| TEXAS INSTRUMENTS INCORPORATED
| Standard Linear and Logic Group
| IBIS Model of SN74ALVCH16646
| 16 BIT BUS TRANSCEIVER AND REGISTER WITH 3-STATE OUTPUTS
| This file contains package information for the following:
|  SSOP 56-pin (DL) package as [Component] ALVCH16646_DL
|  TSSOP 56-pin (DGG) package as [Component] ALVCH16646_DGG
|  TVSOP 56-pin (DGV) package as [Component] ALVCH16646_DGV
| This device can be powered at the following Vccs:
|  2.5 volt Vcc
|  3.3 volt Vcc
|  1.8 volt Vcc
| This file provides unique models under the [Model Selector] for each Vcc.
| For operation at a specific Vcc, select the appropriate model after each
| [Model Selector] keyword.
[IBIS Ver]   3.2
[Comment char]  |_char
[File Name]   sn74alvch16646.ibs
[File Rev]   1.1 | a_die
[Date]   October 1, 2001
[Source]   Data created from TI-SPICE simulations at TI-SLL.
[Notes]   The following is an IBIS list for the ALVCH16646.
   Please contact sllibis@ti.com with questions and
   comments concerning SLL IBIS models.
   This IBIS model is created from a BA (back annotated netlist
   Non-Convergence in the following files:
   gc_alvch16646_noe_33, extrapolated from 0.5 V plus
   gc_alvch16646_dir_25, extrapolated from 0.525 V plus
   Non-Convergence in the following files:
[Disclaimer] Property of Texas Instruments Incorporated.  Unauthorized
   reproduction and/or distribution is strictly prohibited.
   This product is protected under copyright law.
   Created  2001, (C) Copyright  2001, Texas Instruments
   Incorporated, All Rights Reserved
   UNLESS THERE IS A SIGNED, WRITTEN AGREEMENT TO THE
   CONTRARY, TEXAS INSTRUMENTS (TI) IS PROVIDING THE IBIS
   MODELS  AND WITHOUT ANY WARRANTY, EXPRESSED OR
   IMPLIED.  TI assumes no liability for:
   1) the accuracy of the IBIS models provided to your
   company;
   2) the proper functioning of these IBIS Models in your
   design or for any resulting applications; or
   3) infringement of patents, copyrights or intellectual
   property rights resulting from your use of these IBIS
   models.
   TI provides IBIS Models as a service to our customers.
   You and your company shall not distribute, sell or give
   these models to anyone else without prior written
   permission from TI.
   TI reserves the right to make changes to our products or
   to discontinue any semiconductor product or service
   without notice, and advises our customers to obtain the
   latest version of relevant information to verify, before
   placing orders, that the information being relied on is
   current.
   Please be aware that your receipt and use of the IBIS
   information provided shall serve as acceptance of these
   terms and conditions.  If you do not accept these terms,
   you should return or destroy the IBIS models and any
   other accompanying information immediately.
| Component ALVCH16646_DL 56-pin SSOP
[Component]   ALVCH16646_DL
[Manufacturer]   Texas Instruments, Inc.
[Package]
|   typ   min   max
R_pkg   5.500e-02   4.800e-02   6.700e-02
L_pkg   6.539e-09   4.802e-09   9.746e-09
C_pkg   1.880e-13   7.600e-14   5.170e-13
[Pin]   signal_name   model_name   R_pin   L_pin   C_pin
1   1DIR   ALVCH16646_DIR   6.400e-02   9.646e-09   5.130e-13
2   1CLKAB   ALVCH16646_CLK   5.900e-02   8.723e-09   2.700e-13
3   1SAB   ALVCH16646_STORE   5.900e-02   8.139e-09   2.230e-13
4   GND   GND   5.600e-02   7.554e-09   2.010e-13
5   1A1   ALVCH16646_IO   5.400e-02   6.991e-09   1.950e-13
6   1A2   ALVCH16646_IO   5.300e-02   6.659e-09   2.020e-13
7   VCC   POWER   5.500e-02   6.321e-09   2.070e-13
8   1A3   ALVCH16646_IO   5.500e-02   5.942e-09   1.330e-13
9   1A4   ALVCH16646_IO   5.700e-02   5.767e-09   1.320e-13
10   1A5   ALVCH16646_IO   5.400e-02   5.459e-09   1.210e-13
11   GND   GND   5.100e-02   5.224e-09   1.400e-13
12   1A6   ALVCH16646_IO   4.800e-02   5.088e-09   1.260e-13
13   1A7   ALVCH16646_IO   5.000e-02   5.021e-09   9.600e-14
14   1A8   ALVCH16646_IO   5.100e-02   4.802e-09   7.600e-14
15   2A1   ALVCH16646_IO   5.100e-02   4.803e-09   7.600e-14
16   2A2   ALVCH16646_IO   5.000e-02   5.021e-09   9.600e-14
17   2A3   ALVCH16646_IO   4.800e-02   5.088e-09   1.260e-13
18   GND   GND   5.100e-02   5.224e-09   1.400e-13
19   2A4   ALVCH16646_IO   5.400e-02   5.459e-09   1.210e-13
20   2A5   ALVCH16646_IO   5.700e-02   5.768e-09   1.330e-13
21   2A6   ALVCH16646_IO   5.500e-02   5.942e-09   1.330e-13
22   VCC   POWER   5.500e-02   6.320e-09   2.060e-13
23   2A7   ALVCH16646_IO   5.300e-02   6.659e-09   2.030e-13
24   2A8   ALVCH16646_IO   5.400e-02   6.991e-09   1.960e-13
25   GND   GND   5.600e-02   7.554e-09   2.010e-13
26   2SAB   ALVCH16646_STORE   5.900e-02   8.139e-09   2.230e-13
27   2CLKAB   ALVCH16646_CLK   5.900e-02   8.727e-09   2.700e-13
28   2DIR   ALVCH16646_DIR   6.700e-02   9.746e-09   5.170e-13
29   2NOE   ALVCH16646_NOE   6.300e-02   9.630e-09   5.110e-13
30   2CLKBA   ALVCH16646_CLK   6.000e-02   8.751e-09   2.710e-13
31   2SBA   ALVCH16646_STORE   6.000e-02   8.184e-09   2.250e-13
32   GND   GND   5.600e-02   7.543e-09   2.000e-13
33   2B8   ALVCH16646_IO   5.400e-02   7.005e-09   1.960e-13
34   2B7   ALVCH16646_IO   5.600e-02   6.714e-09   2.040e-13
35   VCC   POWER   5.800e-02   6.384e-09   2.080e-13
36   2B6   ALVCH16646_IO   5.700e-02   5.976e-09   1.340e-13
37   2B5   ALVCH16646_IO   5.700e-02   5.743e-09   1.300e-13
38   2B4   ALVCH16646_IO   5.400e-02   5.468e-09   1.190e-13
39   GND   GND   5.500e-02   5.328e-09   1.420e-13
40   2B3   ALVCH16646_IO   5.200e-02   5.189e-09   1.290e-13
41   2B2   ALVCH16646_IO   5.200e-02   5.053e-09   9.600e-14
42   2B1   ALVCH16646_IO   5.100e-02   4.825e-09   7.600e-14
43   1B8   ALVCH16646_IO   5.400e-02   4.896e-09   7.800e-14
44   1B7   ALVCH16646_IO   5.200e-02   5.093e-09   9.700e-14
45   1B6   ALVCH16646_IO   5.100e-02   5.179e-09   1.280e-13
46   GND   GND   5.400e-02   5.314e-09   1.420e-13
47   1B5   ALVCH16646_IO   5.500e-02   5.511e-09   1.210e-13
48   1B4   ALVCH16646_IO   5.700e-02   5.771e-09   1.310e-13
49   1B3   ALVCH16646_IO   5.600e-02   5.957e-09   1.330e-13
50   VCC   POWER   5.500e-02   6.320e-09   2.060e-13
51   1B2   ALVCH16646_IO   5.200e-02   6.621e-09   2.000e-13
52   1B1   ALVCH16646_IO   5.300e-02   6.973e-09   1.950e-13
53   GND   GND   5.700e-02   7.571e-09   2.020e-13
54   1SBA   ALVCH16646_STORE   5.700e-02   8.097e-09   2.220e-13
55   1CLKBA   ALVCH16646_CLK   5.900e-02   8.723e-09   2.710e-13
56   1NOE   ALVCH16646_NOE   6.100e-02   9.560e-09   5.090e-13
| Component ALVCH16646_DGG 56-pin TSSOP
[Component]   ALVCH16646_DGG
[Manufacturer]   Texas Instruments, Inc.
[Package]
|   typ   min   max
R_pkg   4.500e-02   3.500e-02   6.200e-02
L_pkg   3.324e-09   2.403e-09   5.094e-09
C_pkg   5.640e-13   3.410e-13   9.140e-13
[Pin]   signal_name   model_name   R_pin   L_pin   C_pin
1   1DIR   ALVCH16646_DIR   6.200e-02   5.094e-09   8.560e-13
2   1CLKAB   ALVCH16646_CLK   6.100e-02   4.621e-09   9.020e-13
3   1SAB   ALVCH16646_STORE   6.000e-02   4.316e-09   8.020e-13
4   GND   GND   5.900e-02   3.968e-09   6.980e-13
5   1A1   ALVCH16646_IO   5.700e-02   3.716e-09   6.490e-13
6   1A2   ALVCH16646_IO   4.200e-02   3.517e-09   6.520e-13
7   VCC   POWER   4.100e-02   3.160e-09   5.700e-13
8   1A3   ALVCH16646_IO   3.900e-02   2.981e-09   4.820e-13
9   1A4   ALVCH16646_IO   3.900e-02   2.809e-09   4.470e-13
10   1A5   ALVCH16646_IO   3.800e-02   2.715e-09   4.090e-13
11   GND   GND   4.100e-02   2.675e-09   3.910e-13
12   1A6   ALVCH16646_IO   3.900e-02   2.536e-09   3.660e-13
13   1A7   ALVCH16646_IO   3.900e-02   2.457e-09   3.480e-13
14   1A8   ALVCH16646_IO   3.800e-02   2.411e-09   3.530e-13
15   2A1   ALVCH16646_IO   3.900e-02   2.456e-09   3.550e-13
16   2A2   ALVCH16646_IO   3.900e-02   2.471e-09   3.490e-13
17   2A3   ALVCH16646_IO   4.000e-02   2.580e-09   3.700e-13
18   GND   GND   3.800e-02   2.651e-09   3.890e-13
19   2A4   ALVCH16646_IO   3.800e-02   2.739e-09   4.110e-13
20   2A5   ALVCH16646_IO   3.900e-02   2.838e-09   4.490e-13
21   2A6   ALVCH16646_IO   3.800e-02   2.988e-09   4.840e-13
22   VCC   POWER   3.800e-02   3.105e-09   5.640e-13
23   2A7   ALVCH16646_IO   4.000e-02   3.427e-09   6.380e-13
24   2A8   ALVCH16646_IO   5.600e-02   3.654e-09   6.410e-13
25   GND   GND   5.700e-02   3.932e-09   7.000e-13
26   2SAB   ALVCH16646_STORE   5.800e-02   4.257e-09   8.060e-13
27   2CLKAB   ALVCH16646_CLK   5.700e-02   4.580e-09   9.140e-13
28   2DIR   ALVCH16646_DIR   5.900e-02   5.038e-09   8.610e-13
29   2NOE   ALVCH16646_NOE   6.000e-02   5.058e-09   8.580e-13
30   2CLKBA   ALVCH16646_CLK   5.600e-02   4.543e-09   9.040e-13
31   2SBA   ALVCH16646_STORE   5.700e-02   4.240e-09   8.030e-13
32   GND   GND   5.700e-02   3.929e-09   7.000e-13
33   2B8   ALVCH16646_IO   5.600e-02   3.616e-09   6.370e-13
34   2B7   ALVCH16646_IO   3.700e-02   3.368e-09   6.400e-13
35   VCC   POWER   3.600e-02   3.024e-09   5.630e-13
36   2B6   ALVCH16646_IO   3.500e-02   2.876e-09   4.740e-13
37   2B5   ALVCH16646_IO   3.500e-02   2.745e-09   4.440e-13
38   2B4   ALVCH16646_IO   3.700e-02   2.683e-09   4.050e-13
39   GND   GND   3.800e-02   2.603e-09   3.820e-13
40   2B3   ALVCH16646_IO   3.800e-02   2.510e-09   3.620e-13
41   2B2   ALVCH16646_IO   3.600e-02   2.412e-09   3.410e-13
42   2B1   ALVCH16646_IO   3.800e-02   2.416e-09   3.490e-13
43   1B8   ALVCH16646_IO   3.700e-02   2.403e-09   3.490e-13
44   1B7   ALVCH16646_IO   3.700e-02   2.429e-09   3.410e-13
45   1B6   ALVCH16646_IO   3.600e-02   2.482e-09   3.580e-13
46   GND   GND   3.700e-02   2.615e-09   3.810e-13
47   1B5   ALVCH16646_IO   3.500e-02   2.669e-09   4.020e-13
48   1B4   ALVCH16646_IO   3.600e-02   2.763e-09   4.420e-13
49   1B3   ALVCH16646_IO   3.600e-02   2.942e-09   4.780e-13
50   VCC   POWER   3.500e-02   3.053e-09   5.640e-13
51   1B2   ALVCH16646_IO   3.600e-02   3.409e-09   6.410e-13
52   1B1   ALVCH16646_IO   5.800e-02   3.698e-09   6.410e-13
53   GND   GND   5.900e-02   3.975e-09   6.970e-13
54   1SBA   ALVCH16646_STORE   6.100e-02   4.327e-09   8.020e-13
55   1CLKBA   ALVCH16646_CLK   6.100e-02   4.624e-09   9.050e-13
56   1NOE   ALVCH16646_NOE   6.000e-02   5.063e-09   8.580e-13
| Component ALVCH16646_DGV 56-pin TVSOP
[Component]   ALVCH16646_DGV
[Manufacturer]   Texas Instruments, Inc.
[Package]
|   typ   min   max
R_pkg   6.300e-02   5.000e-02   8.600e-02
L_pkg   2.945e-09   2.392e-09   3.938e-09
C_pkg   3.910e-13   2.710e-13   5.880e-13
[Pin]   signal_name   model_name   R_pin   L_pin   C_pin
1   1DIR   ALVCH16646_DIR   6.800e-02   3.933e-09   5.880e-13
2   1CLKAB   ALVCH16646_CLK   6.800e-02   3.569e-09   5.860e-13
3   1SAB   ALVCH16646_STORE   7.600e-02   3.464e-09   5.150e-13
4   GND   GND   8.600e-02   3.451e-09   4.580e-13
5   1A1   ALVCH16646_IO   8.200e-02   3.278e-09   4.260e-13
6   1A2   ALVCH16646_IO   7.700e-02   3.143e-09   3.870e-13
7   VCC   POWER   6.900e-02   2.971e-09   4.010e-13
8   1A3   ALVCH16646_IO   5.000e-02   2.787e-09   3.790e-13
9   1A4   ALVCH16646_IO   5.100e-02   2.686e-09   3.200e-13
10   1A5   ALVCH16646_IO   5.200e-02   2.607e-09   3.160e-13
11   GND   GND   5.300e-02   2.497e-09   2.970e-13
12   1A6   ALVCH16646_IO   5.400e-02   2.438e-09   2.920e-13
13   1A7   ALVCH16646_IO   5.500e-02   2.412e-09   2.860e-13
14   1A8   ALVCH16646_IO   5.500e-02   2.400e-09   2.730e-13
15   2A1   ALVCH16646_IO   5.500e-02   2.402e-09   2.730e-13
16   2A2   ALVCH16646_IO   5.400e-02   2.398e-09   2.840e-13
17   2A3   ALVCH16646_IO   5.400e-02   2.407e-09   2.890e-13
18   GND   GND   5.300e-02   2.448e-09   2.930e-13
19   2A4   ALVCH16646_IO   5.200e-02   2.548e-09   3.110e-13
20   2A5   ALVCH16646_IO   5.100e-02   2.623e-09   3.160e-13
21   2A6   ALVCH16646_IO   5.000e-02   2.725e-09   3.700e-13
22   VCC   POWER   6.500e-02   2.903e-09   3.940e-13
23   2A7   ALVCH16646_IO   7.300e-02   3.086e-09   3.870e-13
24   2A8   ALVCH16646_IO   8.200e-02   3.272e-09   4.280e-13
25   GND   GND   8.200e-02   3.394e-09   4.570e-13
26   2SAB   ALVCH16646_STORE   7.100e-02   3.374e-09   5.080e-13
27   2CLKAB   ALVCH16646_CLK   6.900e-02   3.572e-09   5.810e-13
28   2DIR   ALVCH16646_DIR   6.900e-02   3.937e-09   5.740e-13
29   2NOE   ALVCH16646_NOE   6.900e-02   3.923e-09   5.690e-13
30   2CLKBA   ALVCH16646_CLK   6.800e-02   3.546e-09   5.740e-13
31   2SBA   ALVCH16646_STORE   7.400e-02   3.422e-09   5.180e-13
32   GND   GND   8.100e-02   3.395e-09   4.680e-13
33   2B8   ALVCH16646_IO   8.000e-02   3.255e-09   4.310e-13
34   2B7   ALVCH16646_IO   7.100e-02   3.063e-09   3.860e-13
35   VCC   POWER   6.100e-02   2.878e-09   3.900e-13
36   2B6   ALVCH16646_IO   5.000e-02   2.709e-09   3.640e-13
37   2B5   ALVCH16646_IO   5.100e-02   2.607e-09   3.110e-13
38   2B4   ALVCH16646_IO   5.100e-02   2.532e-09   3.060e-13
39   GND   GND   5.300e-02   2.440e-09   2.890e-13
40   2B3   ALVCH16646_IO   5.300e-02   2.399e-09   2.860e-13
41   2B2   ALVCH16646_IO   5.400e-02   2.392e-09   2.820e-13
42   2B1   ALVCH16646_IO   5.500e-02   2.399e-09   2.710e-13
43   1B8   ALVCH16646_IO   5.500e-02   2.395e-09   2.710e-13
44   1B7   ALVCH16646_IO   5.500e-02   2.403e-09   2.830e-13
45   1B6   ALVCH16646_IO   5.400e-02   2.421e-09   2.880e-13
46   GND   GND   5.300e-02   2.472e-09   2.920e-13
47   1B5   ALVCH16646_IO   5.100e-02   2.569e-09   3.090e-13
48   1B4   ALVCH16646_IO   5.100e-02   2.636e-09   3.130e-13
49   1B3   ALVCH16646_IO   5.000e-02   2.739e-09   3.660e-13
50   VCC   POWER   6.500e-02   2.922e-09   3.900e-13
51   1B2   ALVCH16646_IO   7.200e-02   3.076e-09   3.840e-13
52   1B1   ALVCH16646_IO   8.100e-02   3.249e-09   4.300e-13
53   GND   GND   8.300e-02   3.400e-09   4.550e-13
54   1SBA   ALVCH16646_STORE   7.300e-02   3.421e-09   5.060e-13
55   1CLKBA   ALVCH16646_CLK   6.900e-02   3.579e-09   5.780e-13
56   1NOE   ALVCH16646_NOE   6.900e-02   3.938e-09   5.810e-13
| Model ALVCH16646_STORE
[Model Selector]   ALVCH16646_STORE
ALVCH16646_STORE_25   2.5 volt Vcc
ALVCH16646_STORE_33   3.3 volt Vcc
ALVCH16646_STORE_18   1.8 volt Vcc
| Model ALVCH16646_CLK
[Model Selector]   ALVCH16646_CLK
ALVCH16646_CLK_25   2.5 volt Vcc
ALVCH16646_CLK_33   3.3 volt Vcc
ALVCH16646_CLK_18   1.8 volt Vcc
| Model ALVCH16646_NOE
[Model Selector]   ALVCH16646_NOE
ALVCH16646_NOE_25   2.5 volt Vcc
ALVCH16646_NOE_33   3.3 volt Vcc
ALVCH16646_NOE_18   1.8 volt Vcc
| Model ALVCH16646_DIR
[Model Selector]   ALVCH16646_DIR
ALVCH16646_DIR_25   2.5 volt Vcc
ALVCH16646_DIR_33   3.3 volt Vcc
ALVCH16646_DIR_18   1.8 volt Vcc
| Model ALVCH16646_IO
[Model Selector]   ALVCH16646_IO
ALVCH16646_IO_25   2.5 volt Vcc
ALVCH16646_IO_33   3.3 volt Vcc
ALVCH16646_IO_18   1.8 volt Vcc
| Models and submodels in the file (15): ALVCH16646_STORE_25 (Input), ALVCH16646_STORE_33 (Input), ALVCH16646_STORE_18 (Input), ALVCH16646_CLK_25 (Input), ALVCH16646_CLK_33 (Input), ALVCH16646_CLK_18 (Input), ALVCH16646_NOE_25 (Input), ALVCH16646_NOE_33 (Input), ALVCH16646_NOE_18 (Input), ALVCH16646_DIR_25 (Input), ALVCH16646_DIR_33 (Input), ALVCH16646_DIR_18 (Input), ALVCH16646_IO_25 (I/O), ALVCH16646_IO_33 (I/O), ALVCH16646_IO_18 (I/O)
